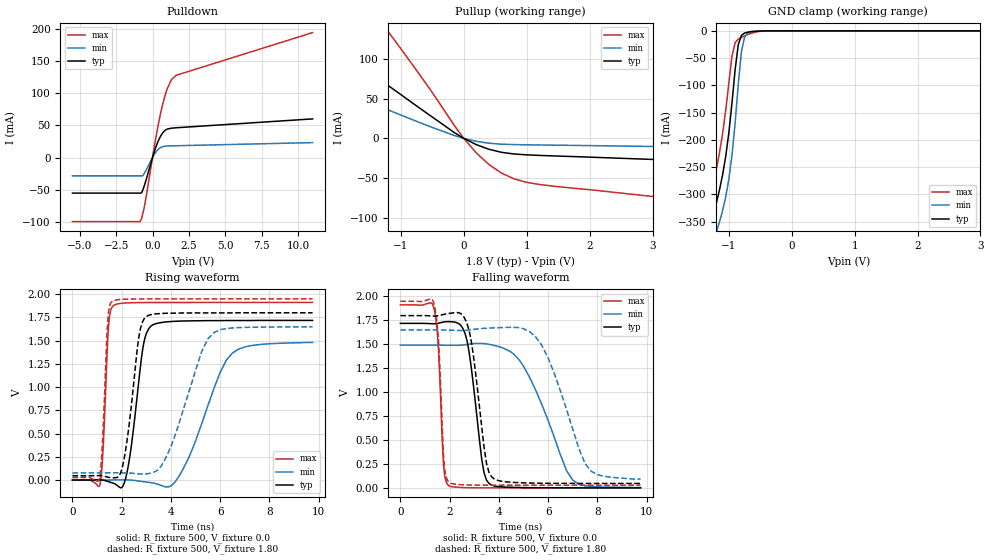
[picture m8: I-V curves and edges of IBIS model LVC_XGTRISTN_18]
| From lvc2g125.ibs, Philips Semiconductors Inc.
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|   Model LVC_XGTRISTN_18
[Model]   LVC_XGTRISTN_18
Model_type   3-state
Polarity   Non-Inverting
Enable   Active-Low
Vmeas =  0.9V
Cref  =  30.0pF
Rref  =  1.0k
Vref  =  0.0V
C_comp   4.00pF   2.90pF   5.15pF
[Model Spec]
| Note: The input and output voltage ratings may be exceeded if the input and
|   output current ratings are observed (please refer to the data sheet)
|   Subparameter   typ   min   max
| Timing Thresholds
Vmeas   0.9   0.825   0.975
|Ambient temperature:   25   85   -40
[Temperature Range]   25   85   -40
[Voltage Range]   1.80V   1.65V   1.95V
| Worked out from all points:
|   slope of the pulldown table from 0 to 0.27 V, typ, clamps not added: 14.4 ohm
|   slope of the pullup table from 0 to 0.27 V, typ, clamps not added: 27.3 ohm
|   GND clamp passes 1 mA (typ) near -0.59 V on its own axis
|   rising waveform, R_fixture 500, V_fixture 0.0: 20-80 % time 456ps typ, 1.24ns min, 183ps max; typ from 0 V to 1.72 V
|   rising waveform, R_fixture 500, V_fixture 1.80: 20-80 % time 448ps typ, 1.15ns min, 180ps max; typ from 0.046 V to 1.8 V
|   falling waveform, R_fixture 500, V_fixture 0.0: 20-80 % time 467ps typ, 1.4ns min, 198ps max; typ from 1.72 V to 0 V
|   falling waveform, R_fixture 500, V_fixture 1.80: 20-80 % time 486ps typ, 1.23ns min, 200ps max; typ from 1.8 V to 0.046 V
|Process Range   nominal   slow   fast
[Pulldown]
| voltage   I(typ)   I(min)   I(max)
-5.5V     -55.08mA   -28.29mA   -99.24mA
-850mV    -55.08mA   -28.29mA   -99.24mA
-750mV    -54.45mA   -28.29mA   -93.93mA
-550mV    -42.65mA   -23.9mA    -75.03mA
-400mV    -31.68mA   -17.82mA   -55.95mA
200mV     14.35mA    7.495mA    27.07mA
500mV     30.88mA    14.78mA    62.72mA
700mV     38.35mA    17.07mA    82.73mA
1V        44.17mA    18.02mA    106.3mA
1.3V      45.72mA    18.26mA    121.1mA
1.6V      46.32mA    18.43mA    127.5mA
11V       60.12mA    23.31mA    194.1mA
[Pullup]
| voltage   I(typ)   I(min)   I(max)
-9.35V    153.8mA    67.09mA    440.4mA
-2.75V    139.8mA    67.09mA    282.4mA
-2.35V    122.3mA    64.83mA    252.3mA
-1.95V    106.4mA    55.63mA    212.6mA
-1.35V    74.64mA    40.41mA    149.5mA
-1.15V    63.51mA    34.17mA    128.6mA
-150mV    7.246mA    3.633mA    16.07mA
200mV     -7.848mA   -3.636mA   -18.36mA
400mV     -13.66mA   -6.01mA    -32.88mA
800mV     -19.57mA   -7.725mA   -50.86mA
1.4V      -21.93mA   -8.426mA   -59.8mA
7.45V     -39.21mA   -14.88mA   -110.8mA
[GND_clamp]
| voltage   I(typ)   I(min)   I(max)
-5.5V     -4.532A    -4.564A    -4.503A
-1.35V    -425.4mA   -472.7mA   -370.6mA
-1.25V    -343.2mA   -392.6mA   -285.9mA
-1.15V    -292.1mA   -350.6mA   -224.3mA
-1.05V    -230mA     -304.3mA   -145.8mA
-950mV    -131.9mA   -227.5mA   -46.26mA
-900mV    -70.6mA    -168.8mA   -21.73mA
-850mV    -25.23mA   -97.39mA   -15.15mA
-800mV    -8.358mA   -38.06mA   -11.92mA
-750mV    -3.999mA   -11.51mA   -9.224mA
-500mV    -375.4uA   -262uA     -895.9uA
5.5V      151.5pA    1.703nA    11.09pA
[Ramp]
| variable   typ   min   max
dV/dt_r   1.031V/455.858ps   888.351mV/1.235ns   1.147V/183.021ps
dV/dt_f   1.053V/486.380ps   935.351mV/1.234ns   1.154V/199.802ps
R_load = 500
[Rising Waveform]
R_fixture   = 500
V_fixture   = 0.0
V_fixture_min = 0.0
V_fixture_max = 0.0
| time   V(typ)   V(min)   V(max)
0s        9.665pV    465.3pV    3.136pV
1.1ns     2.243mV    -143.3uV   -65.15mV
1.45ns    -15.98mV   558.5uV    1.607V
1.7ns     -38.21mV   1.322mV    1.883V
2.2ns     63.39mV    1.764mV    1.907V
2.85ns    1.406V     -16.03mV   1.91V
3.2ns     1.661V     -28.43mV   1.911V
4.3ns     1.71V      30.85mV    1.911V
6.5ns     1.717V     1.368V     1.912V
9.75ns    1.718V     1.481V     1.912V
[Rising Waveform]
R_fixture   = 500
V_fixture   = 1.80
V_fixture_min = 1.65
V_fixture_max = 1.95
| time   V(typ)   V(min)   V(max)
0s        45.81mV    77.33mV    27.35mV
1.1ns     47.26mV    77.34mV    22.43mV
1.45ns    30.64mV    78mV       1.777V
1.6ns     24.71mV    78.21mV    1.92V
2.05ns    167.3mV    77.37mV    1.945V
2.7ns     1.547V     65.94mV    1.949V
3ns       1.76V      66.76mV    1.949V
3.8ns     1.795V     246.6mV    1.95V
5.75ns    1.799V     1.588V     1.95V
9.75ns    1.8V       1.649V     1.95V
[Falling Waveform]
R_fixture   = 500
V_fixture   = 0.0
V_fixture_min = 0.0
V_fixture_max = 0.0
| time   V(typ)   V(min)   V(max)
0s        1.719V     1.492V     1.912V
1.35ns    1.715V     1.492V     1.889V
1.55ns    1.721V     1.491V     1.429V
1.75ns    1.733V     1.491V     244.3mV
1.95ns    1.737V     1.49V      26.3mV
2.7ns     1.543V     1.498V     1.952mV
3.6ns     46.14mV    1.5V       55.7uV
5ns       2.947mV    1.27V      -13.23uV
7ns       100.6uV    81.26mV    -1.362uV
9.75ns    -22.21uV   3.051mV    -49.37nV
[Falling Waveform]
R_fixture   = 500
V_fixture   = 1.80
V_fixture_min = 1.65
V_fixture_max = 1.95
| time   V(typ)   V(min)   V(max)
0s        1.8V       1.65V      1.95V
1.35ns    1.795V     1.65V      1.938V
1.55ns    1.799V     1.65V      1.53V
1.8ns     1.815V     1.649V     192.1mV
2ns       1.824V     1.648V     52.41mV
2.8ns     1.633V     1.651V     29.28mV
3.7ns     117mV      1.671V     27.43mV
5.75ns    47.99mV    1.486V     27.35mV
7.75ns    45.91mV    172.7mV    27.35mV
9.75ns    45.8mV     91.08mV    27.35mV
